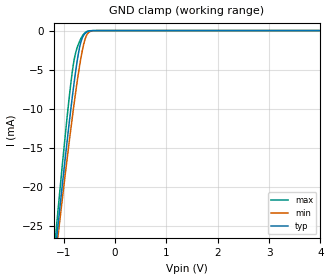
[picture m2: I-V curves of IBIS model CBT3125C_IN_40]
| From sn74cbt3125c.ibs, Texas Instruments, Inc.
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[Model]   CBT3125C_IN_40
Model_type  Input
Vinl=0.8
Vinh=2.0
| variable   typ   min   max
C_comp   2.53pF   1.91pF   3.24pF
[Temperature Range]   40   100   -40
| Ambient temperature   25   85   -40
[Voltage range]   4   4   4
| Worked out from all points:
|   GND clamp passes 1 mA (typ) near -0.64 V on its own axis
[GND Clamp]
| CBT3125C_IN_40
|   Voltage   I(typ)   I(min)   I(max)
-5V       -300.5mA   -278.7mA   -325.7mA
-1.145V   -26.97mA   -28.16mA   -25.27mA
-1.11V    -24.77mA   -26.15mA   -22.81mA
-1.08V    -22.9mA    -24.44mA   -20.72mA
-925mV    -13.57mA   -15.86mA   -10.43mA
-815mV    -7.491mA   -10.15mA   -4.404mA
-765mV    -5.031mA   -7.723mA   -2.745mA
-685mV    -1.94mA    -4.222mA   -1.277mA
-610mV    -563.5uA   -1.689mA   -431.8uA
-550mV    -185.4uA   -533.6uA   -116.2uA
-410mV    -6.399uA   -14.08uA   -1.367uA
4V        94.31pA    243pA      55.56pA
